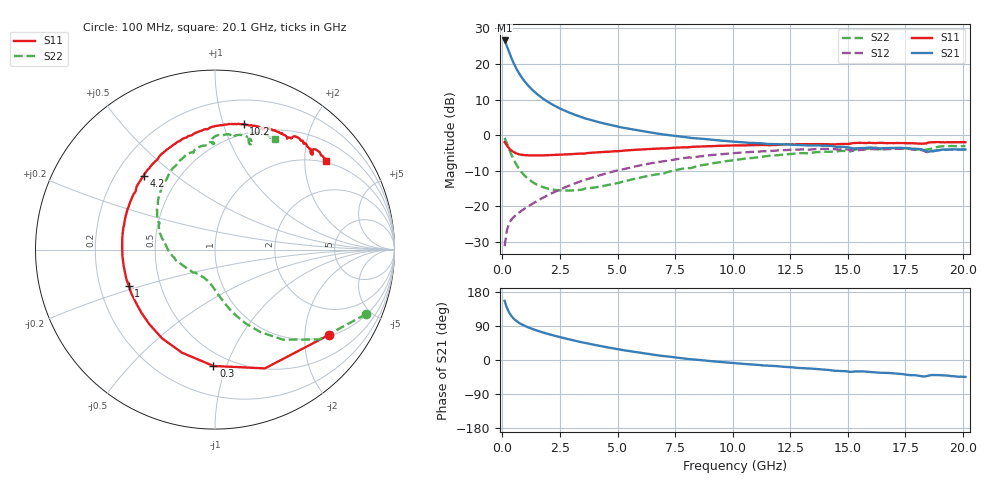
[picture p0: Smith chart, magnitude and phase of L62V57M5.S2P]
!  Infineon Technologies AG
! BFR380L3 , PF131585-7, No.6, Th 09.10.01, soldered on pcb-board, measured with PP GSG850
!  Vce=2.5 V,  Ic=7.5 mA
! Common Emitter S-Parameters:  15. November 2001
#  GHz  S  MA  R  50
! f  S11  S21  S12  S22
! GHz  Mag  Ang  Mag  Ang  Mag  Ang  Mag  Ang
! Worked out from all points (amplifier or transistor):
!   201 points, 100 MHz to 20.1 GHz, reference 50 ohm
!   highest |S21| = 26.6 dB at 100 MHz (marker M1)
!   |S21| within 3 dB of that: start of sweep to 280 MHz
!   unconditionally stable (mu >= 1): 1.996 GHz to 4.614 GHz
!   at 3.4 GHz: K = 1.03, MAG = 7.9 dB, |S12| = -13.0 dB
!   at 10.1 GHz: K = 0.95, MSG = 1.6 dB, |S12| = -5.1 dB
!   at 20.1 GHz: K = 0.99, MSG = 0.0 dB, |S12| = -4.1 dB
!   S11 on the Smith chart (normalised r, x): 100 MHz: 1.03, -2.64; 300 MHz: 0.40, -0.90; 1 GHz: 0.33, -0.18; 4.2 GHz: 0.32, +0.39; 10.2 GHz: 0.41, +1.17; 20.1 GHz: 0.96, +2.55
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0.1  0.7931 -36.9  21.4 156.1  0.02739 70.6  0.9154 -23.1
0.2  0.7178 -67.2  17.81 137.7  0.04639 59.3  0.7672 -40.8
0.3  0.6483 -90.7  14.55 124.9  0.05791 52.1  0.6299 -52.8
0.4  0.6033 -107.7  12.03 115.7  0.06524 48.2  0.5241 -61.2
0.5  0.5758 -120.8  10.14 108.8  0.07097 46.6  0.4468 -67.3
0.6  0.5538 -131.3  8.73 103.6  0.07587 46.0  0.3892 -72.0
0.7  0.5401 -139.5  7.643 99.2  0.08024 46.1  0.3451 -75.8
0.8  0.5302 -146.5  6.782 95.4  0.0847 46.8  0.3112 -79.0
1  0.5214 -157.3  5.535 89.3  0.09367 48.1  0.2632 -84.2
1.2  0.517 -165.7  4.672 84.3  0.1031 49.5  0.2316 -88.8
1.4  0.5163 -172.8  4.046 79.8  0.1126 50.9  0.2097 -93.0
1.9  0.52 173.5  3.046 70.2  0.1386 53.0  0.1796 -102.6
2.6  0.5315 159.2  2.286 58.9  0.1772 53.8  0.1666 -116.2
3.5  0.5483 144.0  1.757 46.2  0.2298 52.0  0.1719 -132.3
4.2  0.5723 134.1  1.515 37.6  0.2701 49.6  0.1881 -146.5
5.2  0.5999 121.7  1.275 26.4  0.3283 44.0  0.2207 -162.6
6.8  0.6445 104.2  1.043 11.8  0.4202 34.7  0.2829 171.2
10.1  0.7146 78.0  0.8065 -8.5  0.5583 13.0  0.447 132.5
10.2  0.7167 77.2  0.8002 -8.9  0.5607 12.3  0.451 131.3
13.5  0.7443 60.1  0.7149 -23.2  0.6308 -8.7  0.5667 101.4
16.8  0.7716 47.9  0.6595 -34.3  0.6353 -25.1  0.6514 78.7
20.1  0.7921 38.4  0.6265 -44.7  0.6254 -38.9  0.702 61.8
